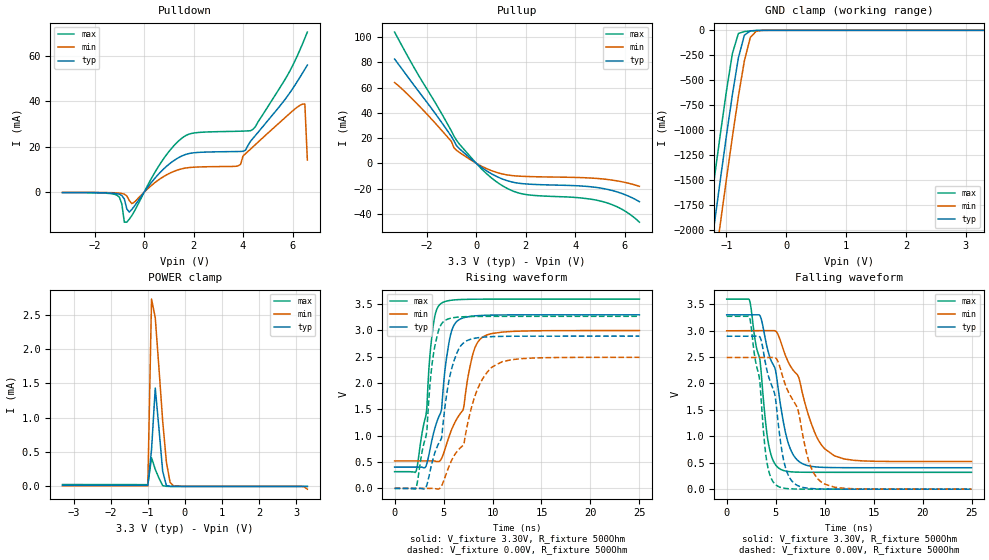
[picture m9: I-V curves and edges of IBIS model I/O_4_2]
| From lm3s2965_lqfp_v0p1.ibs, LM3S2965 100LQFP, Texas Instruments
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[Model]   I/O_4_2
Model_type   I/O
Vinl = 1.26
Vinh = 2.04
Vmeas = 1.65
| variable   typ   min   max
C_comp   9.739pF   9.739pF   9.739pF
[Model Spec]
Vinh+   1.91   1.78   2.04
Vinh-   1.90   1.76   2.03
Vinl+   1.40   1.27   1.54
Vinl-   1.39   1.26   1.53
| variable   typ   min   max
[Temperature Range]  25   85   -40
[Voltage Range]   3.3V   3.0V   3.6V
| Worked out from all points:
|   slope of the pulldown table from 0 to 0.495 V, typ, clamps not added: 71.5 ohm
|   slope of the pullup table from 0 to 0.495 V, typ, clamps not added: 71.6 ohm
|   GND clamp passes 1 mA (typ) near -0.48 V on its own axis
|   POWER clamp passes 1 mA (typ) near -0.73 V on its own axis
|   falling waveform, V_fixture 3.30V, R_fixture 500Ohm: 20-80 % time 2.03ns typ, 3.06ns min, 1.36ns max; typ from 3.3 V to 0.405 V
|   rising waveform, V_fixture 3.30V, R_fixture 500Ohm: 20-80 % time 1.62ns typ, 2.31ns min, 1.11ns max; typ from 0.405 V to 3.3 V
|   falling waveform, V_fixture 0.00V, R_fixture 500Ohm: 20-80 % time 1.75ns typ, 2.48ns min, 1.21ns max; typ from 2.89 V to 0 V
|   rising waveform, V_fixture 0.00V, R_fixture 500Ohm: 20-80 % time 1.94ns typ, 2.99ns min, 1.26ns max; typ from 0 V to 2.89 V
[Pulldown]
|  Voltage   I(typ)   I(min)   I(max)
-3.3V     -128.3uA   -72.81uA   -182.3uA
-1.1V     -636.5uA   -293.8uA   -1.284mA
-800mV    -2.996mA   -835.1uA   -13.2mA
-700mV    -7.355mA   -1.607mA   -13.16mA
-500mV    -7.628mA   -5mA       -10.33mA
700mV     9.309mA    6.304mA    13.37mA
1.6V      16.33mA    10.51mA    24.41mA
3.8V      17.94mA    11.61mA    26.87mA
4.4V      23.7mA     20mA       27.72mA
6.4V      52.42mA    38.8mA     65.24mA
6.5V      54.21mA    38.87mA    67.86mA
6.6V      56.01mA    14.21mA    70.56mA
[Pullup]
|  Voltage   I(typ)   I(min)   I(max)
-3.3V     82.57mA    63.94mA    103.9mA
-1.8V     43.25mA    34.86mA    52.68mA
-1V       21.14mA    17.2mA     25.44mA
-900mV    17.77mA    12.26mA    21.52mA
-800mV    14.06mA    10.32mA    18.34mA
100mV     -1.553mA   -1.117mA   -2.117mA
700mV     -9.22mA    -6.424mA   -12.9mA
1.3V      -14.07mA   -9.367mA   -20.37mA
1.9V      -16.2mA    -10.35mA   -24.39mA
5.2V      -20.26mA   -12.6mA    -30.84mA
5.9V      -24.02mA   -14.69mA   -36.54mA
6.6V      -30.45mA   -18.28mA   -46.68mA
[GND Clamp]
|  Voltage   I(typ)   I(min)   I(max)
-3.3V     -11.72A    -12.12A    -11.3A
-1.4V     -2.845A    -3.285A    -2.387A
-1.3V     -2.39A     -2.831A    -1.93A
-1.2V     -1.938A    -2.38A     -1.478A
-1.1V     -1.494A    -1.934A    -1.036A
-1V       -1.059A    -1.496A    -610.6mA
-900mV    -645mA     -1.069A    -232.9mA
-800mV    -277.1mA   -664.4mA   -31.59mA
-700mV    -48.56mA   -306.6mA   -12.09mA
-600mV    -5.558mA   -70.2mA    -6.272mA
-500mV    -1.167mA   -7.88mA    -2.167mA
3.3V      2.282nA    3.101uA    451.3pA
[POWER Clamp]
|  Voltage   I(typ)   I(min)   I(max)
-3.3V     15.18uA    8.315uA    27.48uA
-1V       14.14uA    7.74uA     25.63uA
-900mV    536uA      2.726mA    416.7uA
-800mV    1.43mA     2.454mA    247.6uA
-700mV    840.7uA    1.719mA    119.9uA
-600mV    221.2uA    951.5uA    11.58uA
-500mV    12.35uA    355.6uA    955.3nA
-400mV    305.2nA    58.59uA    44.3nA
-300mV    9.515nA    3.101uA    1.472nA
3.1V      1.302nA    -112.7nA   143.5pA
3.2V      1.207nA    -2.287uA   131.7pA
3.3V      -104.8pA   -40.34uA   119.2pA
[Ramp]
| variable   typ   min   max
dV/dt_f   1.73/2.03n   1.48/3.06n   1.97/1.36n
dV/dt_r   1.74/1.94n   1.49/2.99n   1.96/1.26n
R_load = 500Ohm
[Falling Waveform]
V_fixture = 3.30V
V_fixture_min = 3.00V
V_fixture_max = 3.60V
R_fixture = 500Ohm
|   Time   V(typ)   V(min)   V(max)
0s        3.297V     2.994V     3.595V
2.3ns     3.297V     2.997V     3.59V
3.4ns     3.283V     2.998V     2.441V
4.3ns     2.559V     2.998V     826.9mV
5.3ns     1.846V     2.901V     400mV
6.1ns     994.8mV    2.482V     339.4mV
6.9ns     620.2mV    2.226V     324.5mV
9.2ns     419.7mV    985.1mV    318.8mV
11ns      407.7mV    630.6mV    318.6mV
25ns      405.4mV    522.4mV    318.5mV
[Rising Waveform]
V_fixture = 3.30V
V_fixture_min = 3.00V
V_fixture_max = 3.60V
R_fixture = 500Ohm
|   Time   V(typ)   V(min)   V(max)
0s        405.4mV    522.4mV    318.5mV
2.2ns     405.4mV    522.4mV    327.6mV
3.2ns     420.5mV    522.4mV    1.383V
4ns       1.067V     522.1mV    3.164V
4.8ns     1.506V     570.5mV    3.521V
5.3ns     2.474V     838.3mV    3.558V
6ns       3.077V     1.194V     3.579V
7ns       3.239V     1.496V     3.59V
9ns       3.287V     2.875V     3.595V
25ns      3.298V     2.999V     3.597V
[Falling Waveform]
V_fixture = 0.00V
V_fixture_min = 0.00V
V_fixture_max = 0.00V
R_fixture = 500Ohm
|   Time   V(typ)   V(min)   V(max)
0s        2.893V     2.49V      3.27V
2.3ns     2.893V     2.491V     3.264V
3.4ns     2.877V     2.491V     2.005V
4.1ns     2.254V     2.491V     517.1mV
5.1ns     1.527V     2.462V     69.45mV
5.7ns     654.7mV    2.142V     23.49mV
6.4ns     225.2mV    1.803V     7.427mV
8.5ns     14.01mV    465.6mV    487.9uV
9.8ns     3.391mV    117.3mV    171.8uV
25ns      17.18uV    28.46uV    11.66uV
[Rising Waveform]
V_fixture = 0.00V
V_fixture_min = 0.00V
V_fixture_max = 0.00V
R_fixture = 500Ohm
|   Time   V(typ)   V(min)   V(max)
0s        186.9uV    3.8mV      10.33uV
2.2ns     29.22uV    789.5uV    11.85mV
3.3ns     69.38mV    374.1uV    1.1V
4ns       612.6mV    -32.31uV   2.589V
4.8ns     961.2mV    50.1mV     3.127V
5.1ns     1.486V     187.8mV    3.184V
6.7ns     2.693V     769.4mV    3.258V
8.4ns     2.859V     1.853V     3.267V
10ns      2.884V     2.312V     3.269V
25ns      2.893V     2.49V      3.269V
